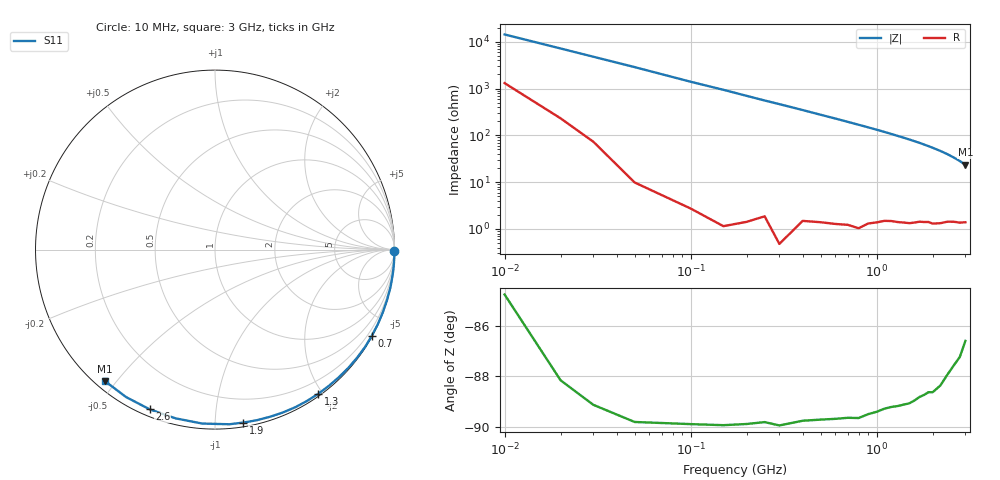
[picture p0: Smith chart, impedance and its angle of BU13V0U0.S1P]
! SIEMENS Small Signal Semiconductors
! BB833
! Si Tuning Diode in SOD323
! VR = 13 V
! S-Parameters:  April  1996
# GHz  S  MA  R  50
!  f  S11
! GHz  MAG  ANG
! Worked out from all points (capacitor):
!   31 points, 10 MHz to 3 GHz, reference 50 ohm
!   read as one part to ground: C = 1.11 pF near 10 MHz
!   lowest |Z| = 23.4 ohm at 3 GHz (marker M1)
!   S11 on the Smith chart (normalised r, x): 10 MHz: open; 700 MHz: 0.02, -3.88; 1.3 GHz: 0.03, -1.94; 1.9 GHz: 0.03, -1.17; 2.6 GHz: 0.03, -0.67; 3 GHz: 0.03, -0.47
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0.01  0.9994 -0.4
0.05  0.9999 -2.0
0.1  0.9999 -4.1
0.2  0.9997 -8.2
0.25  0.9994 -10.3
0.3  0.9998 -12.3
0.4  0.9988 -16.4
0.5  0.9982 -20.6
0.6  0.9977 -24.7
0.7  0.997 -28.9
0.8  0.9966 -33.1
0.9  0.9947 -37.3
1  0.9931 -41.5
1.1  0.991 -45.8
1.2  0.9895 -50.1
1.3  0.9883 -54.5
1.4  0.9869 -58.8
1.5  0.9855 -63.1
1.6  0.9832 -67.5
1.7  0.9805 -71.8
1.8  0.9787 -76.4
1.9  0.9766 -80.8
2  0.9764 -85.3
2.2  0.9719 -94.2
2.4  0.9655 -103.2
2.6  0.9614 -112.3
2.8  0.9594 -121.1
3  0.9553 -129.8
